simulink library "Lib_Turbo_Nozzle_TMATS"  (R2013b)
settings: Solver=ode45  StartTime=0.0  StopTime=10.0  RelTol=1e-3
undefined symbols (not defined in the file or in its folder): iDesign_M, N_EArea_M, N_TArea_M
libraries: Lib_Solve_DataOut_TMATS x2

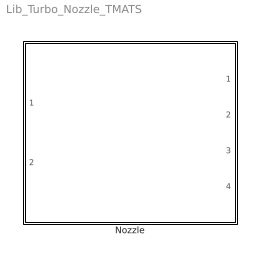
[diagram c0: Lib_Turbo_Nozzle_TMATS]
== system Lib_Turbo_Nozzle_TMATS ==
  Nozzle : Subsystem

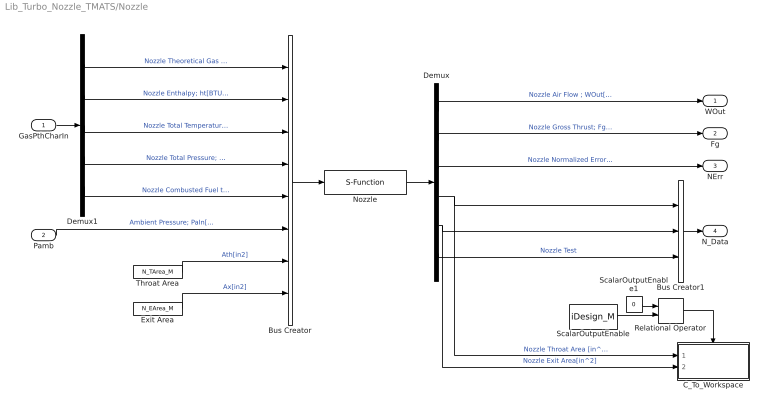
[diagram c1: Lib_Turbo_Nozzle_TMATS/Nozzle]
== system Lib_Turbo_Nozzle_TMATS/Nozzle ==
  GasPthCharIn : Inport
  Pamb : Inport  Port=2
  Bus Creator : BusCreator  Inputs=8
  Bus Creator1 : BusCreator  Inputs=3
  C_To_Workspace : Subsystem
  Demux : Demux  Outputs=6
  Demux1 : Demux  Outputs=5
  Exit Area : Constant  Value=N_EArea_M
  Nozzle : S-Function  FunctionName=Nozzle_TMATS  Parameters=SWType_M, N_FL_M, X_N_FARVec_M, T_N_RtArray_M, Y_N_TtVec_M, T_N_MAP_gammaArray_M, X_N_PEQPaVec_M, T_N_CdThArray_M, T_N_CvArray_M, T_N_CfgArray_M, T_N_TGArray_M, X_N_TtVec2_M, iDesign_M, WDes_M, gcs  EnableBusSupport=off
  Relational Operator : RelationalOperator  Operator===  OutDataTypeStr=boolean
  ScalarOutputEnable : Constant  Value=iDesign_M
  ScalarOutputEnable1 : Constant  Value=0
  Throat Area : Constant  Value=N_TArea_M
  WOut : Outport
  Fg : Outport  Port=2
  NErr : Outport  Port=3
  N_Data : Outport  Port=4
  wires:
  Demux1/4 -> Bus Creator/4  "Nozzle Total Pressure; PtIn[psia]"
  Pamb/1 -> Bus Creator/6  "Ambient Pressure; PaIn[psia]"
  Bus Creator/1 -> Nozzle/1
  Demux/2 -> Fg/1  "Nozzle Gross Thrust; FgOut [lbf]"
  Demux/1 -> WOut/1  "Nozzle Air Flow ; WOut[pps]"
  Nozzle/1 -> Demux/1
  Demux1/3 -> Bus Creator/3  "Nozzle Total Temperature; TtIn[degR]"
  Demux1/5 -> Bus Creator/5  "Nozzle Combusted Fuel to Air Ratio; FARcIn[frac]"
  Demux/5 -> C_To_Workspace/2(Ax), Bus Creator1/2  "Nozzle Exit Area[in^2]"
  GasPthCharIn/1 -> Demux1/1
  Demux1/1 -> Bus Creator/1  "Nozzle Theoretical Gas Flow Input; WIn[pps]"
  Demux/3 -> NErr/1  "Nozzle Normalized Error [frac]"
  Demux1/2 -> Bus Creator/2  "Nozzle Enthalpy; ht[BTU/lbm]"
  Demux/4 -> C_To_Workspace/1(Ath), Bus Creator1/1  "Nozzle Throat Area [in^2]"
  Bus Creator1/1 -> N_Data/1
  ScalarOutputEnable/1 -> Relational Operator/2
  ScalarOutputEnable1/1 -> Relational Operator/1
  Relational Operator/1 -> C_To_Workspace/Enable
  Throat Area/1 -> Bus Creator/7  "Ath[in2]"
  Exit Area/1 -> Bus Creator/8  "Ax[in2]"
  Demux/6 -> Bus Creator1/3  "Nozzle Test"

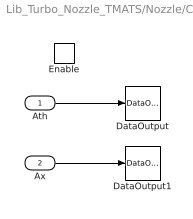
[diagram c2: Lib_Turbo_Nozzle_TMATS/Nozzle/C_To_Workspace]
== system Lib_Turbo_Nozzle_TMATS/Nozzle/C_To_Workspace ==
  Ath : Inport
  Ax : Inport  Port=2
  Enable : EnablePort
  DataOutput : Lib_Solve_DataOut_TMATS/DataOutput  FVar_M=FVar_M  Var_M=AthNm_M  SVar_M=SVar_M
  DataOutput1 : Lib_Solve_DataOut_TMATS/DataOutput  FVar_M=FVar_M  Var_M=AxNm_M  SVar_M=SVar_M
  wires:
  Ath/1 -> DataOutput/1
  Ax/1 -> DataOutput1/1
